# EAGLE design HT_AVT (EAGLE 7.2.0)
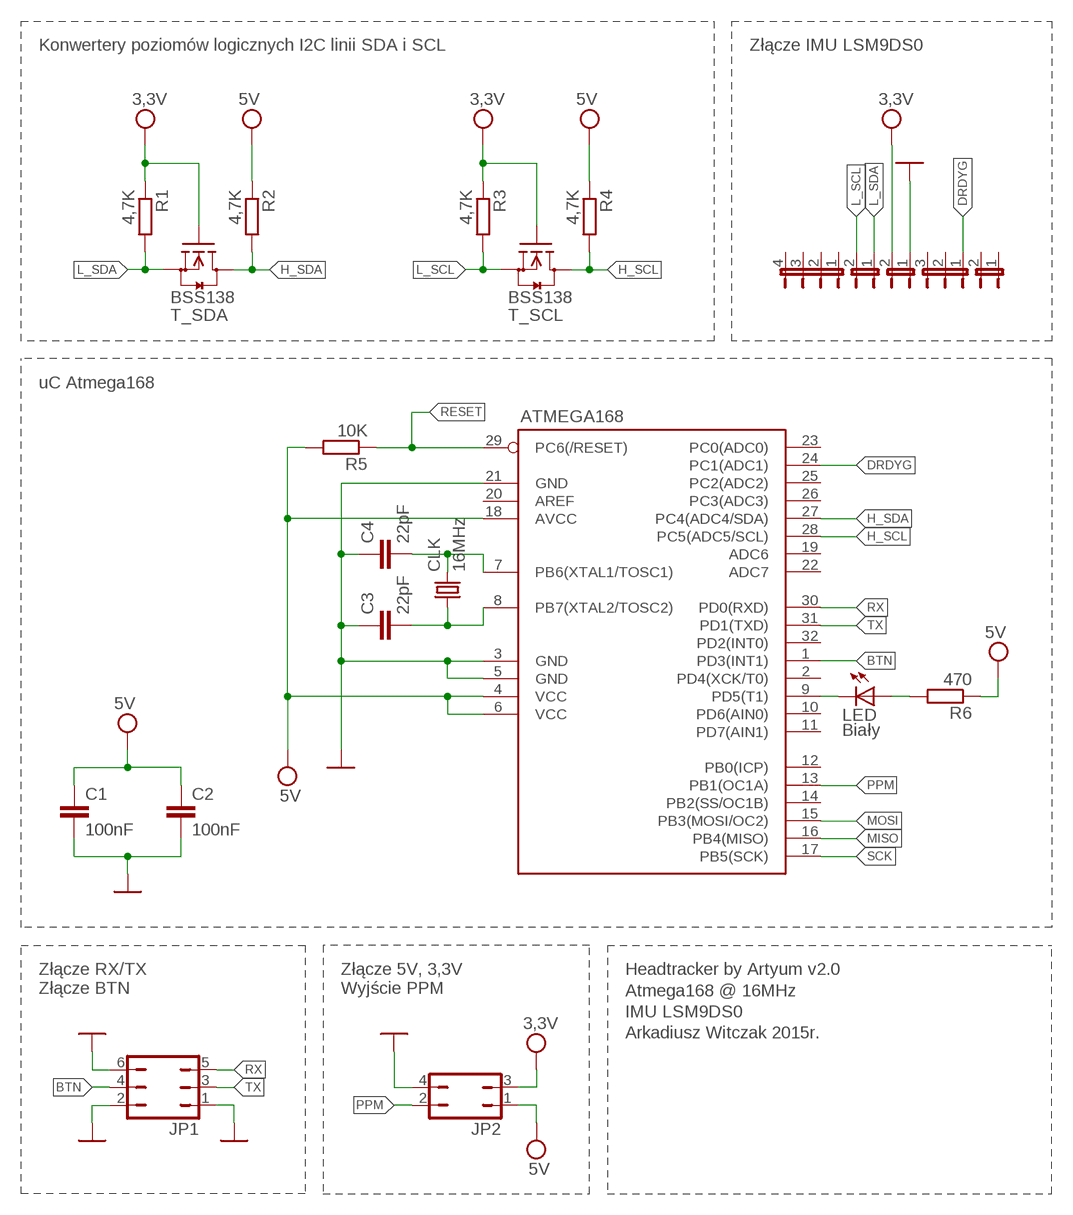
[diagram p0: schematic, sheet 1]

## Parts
ATMEGA168  MEGA8-AI  [TQFP32-08]
C1  100nF  C-EUC0805  [C0805]
C2  100nF  C-EUC0805  [C0805]
C3  22pF  C-EUC0805  [C0805]
C4  22pF  C-EUC0805  [C0805]
CLK  16MHz  CRYSTALHC49U-V  [HC49U-V]
J1  JP1E  [JP1]
J2  JP1E  [JP1]
J3  JP1E  [JP1]
J4  JP2E  [JP2]
J5  JP4E  [JP4]
JP1  JP3Q  [JP3Q]
JP2  JP2Q  [JP2Q]
LED  Biały  LEDCHIPLED_0805  [CHIPLED_0805]
R1  4,7K  R-EU_R0805  [R0805]
R2  4,7K  R-EU_R0805  [R0805]
R3  4,7K  R-EU_R0805  [R0805]
R4  4,7K  R-EU_R0805  [R0805]
R5  10K  R-EU_R0805  [R0805]
R6  470  R-EU_R0805  [R0805]
T_SCL  BSS138  [SOT23]
T_SDA  BSS138  [SOT23]

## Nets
BTN: ATMEGA168.1(PD3(INT1)) JP1.4
DRDYG: ATMEGA168.24(PC1(ADC1)) J4.1
GND: ATMEGA168.3(GND) ATMEGA168.5(GND) ATMEGA168.21(GND) C1.2 C2.2 C3.1 C4.1 J3.1 JP1.1 JP1.2 JP1.6 JP2.4
H_SCL: ATMEGA168.28(PC5(ADC5/SCL)) R4.2 T_SCL.3(D)
H_SDA: ATMEGA168.27(PC4(ADC4/SDA)) R2.2 T_SDA.3(D)
HV: ATMEGA168.4(VCC) ATMEGA168.6(VCC) ATMEGA168.18(AVCC) C1.1 C2.1 JP2.1 R2.1 R4.1 R5.2 R6.1 ; supply symbol labelled 5V
L_SCL: J2.2 R3.2 T_SCL.2(S)
L_SDA: J2.1 R1.2 T_SDA.2(S)
LV: J3.2 JP2.3 R1.1 R3.1 T_SCL.1(G) T_SDA.1(G) ; supply symbol labelled 3,3V
MISO: ATMEGA168.16(PB4(MISO))
MOSI: ATMEGA168.15(PB3(MOSI/OC2))
N$3: ATMEGA168.8(PB7(XTAL2/TOSC2)) C3.2 CLK.1
N$4: ATMEGA168.9(PD5(T1)) LED.C
N$5: ATMEGA168.7(PB6(XTAL1/TOSC1)) C4.2 CLK.2
N$8: LED.A R6.2
PPM: ATMEGA168.13(PB1(OC1A)) JP2.2
RESET: ATMEGA168.29(PC6(/RESET)) R5.1
RX: ATMEGA168.30(PD0(RXD)) JP1.5
SCK: ATMEGA168.17(PB5(SCK))
TX: ATMEGA168.31(PD1(TXD)) JP1.3
Unconnected: ATMEGA168.2(PD4(XCK/T0)) ATMEGA168.10(PD6(AIN0)) ATMEGA168.11(PD7(AIN1)) ATMEGA168.12(PB0(ICP)) ATMEGA168.14(PB2(SS/OC1B)) ATMEGA168.19(ADC6) ATMEGA168.20(AREF) ATMEGA168.22(ADC7) ATMEGA168.23(PC0(ADC0)) ATMEGA168.25(PC2(ADC2)) ATMEGA168.26(PC3(ADC3)) ATMEGA168.32(PD2(INT0)) J1.1 J1.2 J4.2 J4.3 J5.1 J5.2 J5.3 J5.4

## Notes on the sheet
- Konwertery poziomów logicznych I2C linii SDA i SCL | Złącze IMU LSM9DS0
- uC Atmega168
- Złącze RX/TX
  Złącze BTN
- Złącze 5V, 3,3V
  Wyjście PPM
- Headtracker by Artyum v2.0 
  Atmega168 @ 16MHz
  IMU LSM9DS0
  Arkadiusz Witczak 2015r.

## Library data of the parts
ATMEGA168 = atmel:MEGA8: MICROCONTROLLER 8 Kbytes FLASH, 1 kbytes SRAM, 512 bytes EEPROM, USART, 6-channel 10 bit ADC, 2-channel 8 bit ADC Pin compatible with Atmega48, ATMega88, ATMega168 Source: avr.lbr; MPN: ATMEGA8-16AU; OC_FARNELL: 9171371; OC_NEWARK: 73M8863
C1-C4 = rcl:C-EU: CAPACITOR, European symbol
CLK = crystal:CRYSTAL: CRYSTAL; OC_FARNELL: 1666969; OC_NEWARK: unknown
J1-J3 = jumper:JP1E: JUMPER
J4 = jumper:JP2E: JUMPER
J5 = jumper:JP4E: JUMPER
JP1 = jumper:JP3Q: JUMPER
JP2 = jumper:JP2Q: JUMPER
LED = led:LED: LED
R1-R6 = rcl:R-EU_: RESISTOR, European symbol
T_SCL T_SDA = m-pad-2.1:BSS138: Fairchild Semiconductors BSS138 N-Channel Logic Level Enhancement Mode Field Effect Transistor General Description: These N-Channel enhancement mode field effect transistors are produced using Fairchild's proprietary, high cell density, DMOS technology. These products have been designed to minimize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

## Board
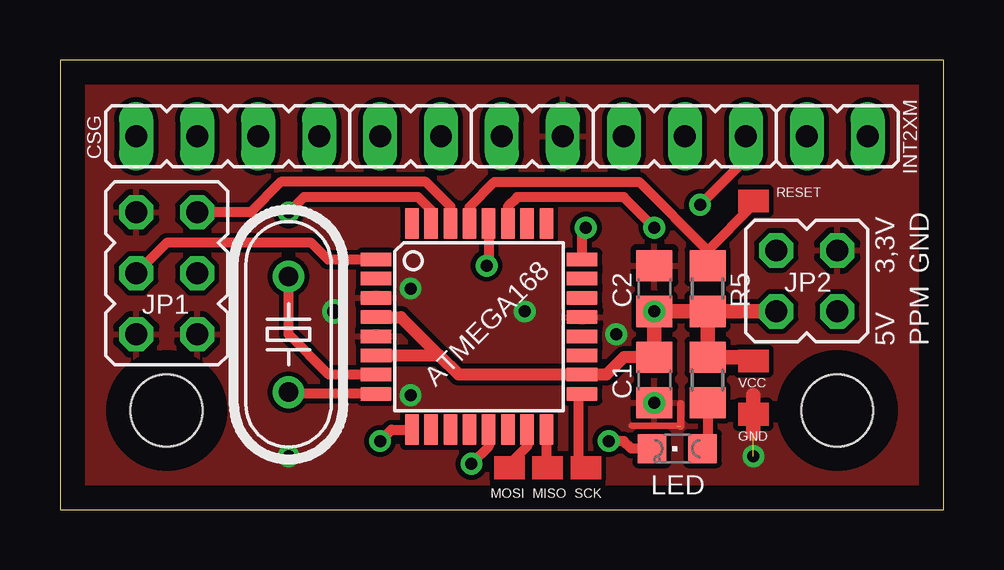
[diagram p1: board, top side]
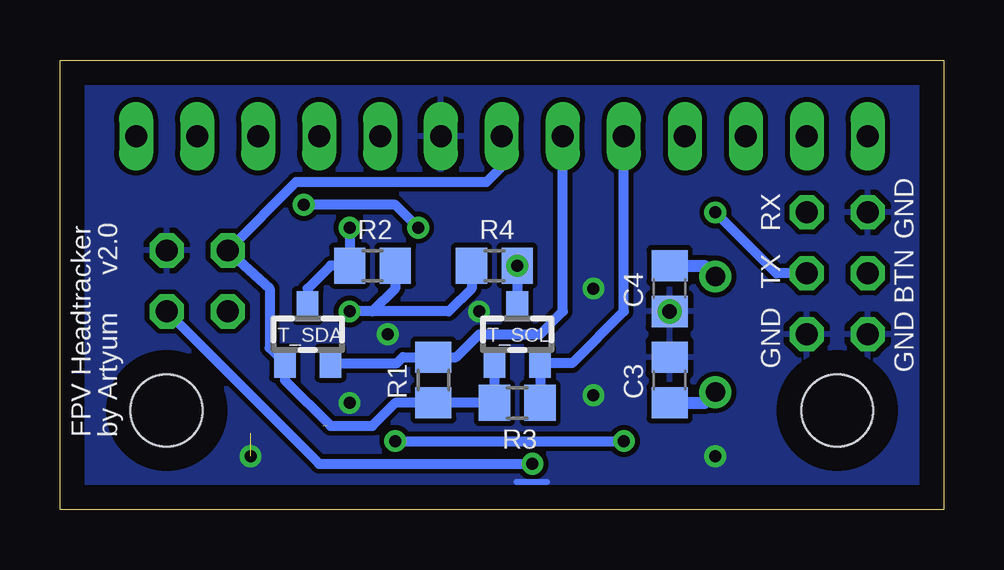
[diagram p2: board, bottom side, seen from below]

Size 36.83 x 18.73 mm. Coordinates in mm from the lower left corner, seen from the top.
Outline: 0,0 36.83,0 36.83,18.73 0,18.73 0,0
Copper layers (1*16): Top 0.035mm / dielectric 1.5mm / Bottom 0.035mm
Design rules "default": minimum track width 10mil, minimum drill 24mil, track to track 8mil, track to pad 8mil, pad to pad 8mil, via to via 8mil, smd to smd 8mil, copper to edge 40mil, drill to drill 8mil, minimum pad ring 10mil, minimum via ring 8mil, stop-mask expansion 4mil, vias tented up to drill 0mil, thermal gap 10mil
Holes 3 mm at 32.38,4.13 4.45,4.13

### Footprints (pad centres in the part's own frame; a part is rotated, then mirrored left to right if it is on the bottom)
TQFP32-08 = smd 1.27 x 0.559: 1 -4.293,2.8; 2 -4.293,2; 3 -4.293,1.2; 4 -4.293,0.4; 5 -4.293,-0.4; 6 -4.293,-1.2; 7 -4.293,-2; 8 -4.293,-2.8; 17 4.293,-2.8; 18 4.293,-2; 19 4.293,-1.2; 20 4.293,-0.4; 21 4.293,0.4; 22 4.293,1.2; 23 4.293,2; 24 4.293,2.8 | smd 0.559 x 1.27: 9 -2.8,-4.293; 10 -2,-4.293; 11 -1.2,-4.293; 12 -0.4,-4.293; 13 0.4,-4.293; 14 1.2,-4.293; 15 2,-4.293; 16 2.8,-4.293; 25 2.8,4.293; 26 2,4.293; 27 1.2,4.293; 28 0.4,4.293; 29 -0.4,4.293; 30 -1.2,4.293; 31 -2,4.293; 32 -2.8,4.293
C0805 = smd 1.3 x 1.5: 1 -0.95,0; 2 0.95,0
HC49U-V = drill 0.813: 1 -2.413,0; 2 2.413,0
JP1 = drill 0.914 long: 1 0,-1.27; 2 0,1.27
JP2 = drill 0.914 long: 1 -2.54,0; 2 0,0; 3 2.54,0
JP4 = drill 0.914 long: 1 -3.81,0; 2 -1.27,0; 3 1.27,0; 4 3.81,0
JP3Q = drill 0.914 octagon: 1 -2.54,-1.27; 2 -2.54,1.27; 3 0,-1.27; 4 0,1.27; 5 2.54,-1.27; 6 2.54,1.27
JP2Q = drill 0.914 octagon: 1 -1.27,-1.27; 2 1.27,-1.27; 3 -1.27,1.27; 4 1.27,1.27
CHIPLED_0805 = smd 1.2 x 1.2: A 0,-1.05; C 0,1.05
R0805 = smd 1.3 x 1.5: 1 -0.95,0; 2 0.95,0
SOT23 = smd 0.9 x 1.2: 1 -0.95,-1.2; 2 0.95,-1.2; 3 0,1.2

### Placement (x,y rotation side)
ATMEGA168  17.46,7.62 0 top
C1  24.77,5.4 270 top
C2  24.77,9.21 90 top
C3  11.43,5.4 270 bottom
C4  11.43,9.21 90 bottom
CLK  9.52,7.3 90 top
J1  32.38,15.56 270 top
J2  14.6,15.56 90 top
J3  19.69,15.56 90 top
J4  26.03,15.56 180 top
J5  6.98,15.56 180 top
JP1  4.45,9.84 90 top
JP2  31.12,9.53 0 top
LED  25.72,2.54 90 top
R1  21.27,5.4 90 bottom
R2  23.81,10.16 180 bottom
R3  17.78,4.45 0 bottom
R4  18.73,10.16 0 bottom
R5  26.99,9.21 270 top
R6  26.99,5.4 270 top
T_SCL  17.78,7.3 0 bottom
T_SDA  26.51,7.3 0 bottom

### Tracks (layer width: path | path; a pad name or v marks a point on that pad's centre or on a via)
BTN
  Top 0.406: ATMEGA168.1 11.17,10.42 10.48,11.11 4.45,11.11 JP1.4
DRDYG  (via drill 0.5)
  Top 0.406: v26.67,12.7 28.57,14.61 J4.1 | ATMEGA168.24 21.76,11.6 v21.91,11.75
  Bottom 0.406: v26.67,12.7 22.86,12.7 v21.91,11.75
GND  (via drill 0.5, 0.6)  (2 unrouted)
  Top 0.279: 25.72,3.49 23.81,3.49
  Top 0.305: 25.87,4.42 25.87,3.47
  Top 0.61: 28.89,4.76 28.89,3.18
  Bottom 0.254: 16.54,1.14 17.81,1.14
  other vias: 23.18,7.3 14.6,4.76 14.6,9.21 11.43,8.25 19.37,8.25 24.77,4.45 20.95,15.56 5.71,7.3 3.18,7.3 3.18,12.38 32.38,10.79 28.89,2.22 9.52,2.22
  pour Bottom: -0.95,19.68 37.78,19.68 37.78,-0.95 -0.95,-0.95
  pour Top: -0.64,19.37 37.46,19.37 37.46,-0.64 -0.64,-0.64
H_SCL  (via drill 0.5)
  Top 0.406: ATMEGA168.28 17.86,10.24 R4.2
  Bottom 0.406: R4.2 T_SCL.3
  other vias: 17.78,10.16
H_SDA  (via drill 0.5)
  Top 0.406: v24.77,11.75 23.49,13.02 19.05,13.02 18.66,12.63 ATMEGA168.27
  Bottom 0.406: v24.77,11.75 24.77,11.43 R2.2 25.56,10.16 26.51,9.21 T_SDA.3
HV  (via drill 0.5)  (1 unrouted)
  Top 0.406: R5.2
  Top 0.508: ATMEGA168.4 14.2,8.02 15.81,6.42 | 15.81,6.42 ATMEGA168.6 | 15.81,6.42 16.6,5.62 ATMEGA168.18 22.77,5.62 23.49,6.35 C1.1
  Top 0.61: JP2.1 R5.2 R6.1 | R5.2 C2.1 | C2.1 C1.1 | R6.1 | R6.1 28.73,6.35
  Bottom 0.406: R2.1 22.86,9.21 23.81,8.25 | R4.1 19.68,9.21 20.64,8.25 23.81,8.25 | 23.81,8.25 C2.1
  other vias: 24.77,8.25
L_SCL
  Bottom 0.406: J2.2 13.34,8.25 15.49,6.1 T_SCL.2 R3.2
L_SDA
  Bottom 0.406: J2.1 15.88,8.25 16.83,7.3 19.37,7.3 20.32,6.35 R1.2 22.54,6.35 22.79,6.1 T_SDA.2
LV
  Bottom 0.406: J3.2 18.42,14.29 19.05,13.65 26.99,13.65 JP2.3 28.1,9.21 28.1,6.74 T_SDA.1 27.46,5.39 25.56,3.49 23.81,3.49 22.86,4.45 R1.1 R3.1 T_SCL.1
MISO
  Top 0.406: ATMEGA168.16 20.26,1.8
MOSI
  Top 0.406: ATMEGA168.15 19.46,2.63 18.73,1.9
N$3
  Top 0.406: ATMEGA168.8 9.59,4.82 CLK.1
  Bottom 0.508: C3.2 9.97,4.45 CLK.1
N$4  (via drill 0.5)
  Top 0.406: v13.34,2.86 13.8,3.33 ATMEGA168.9 | LED.C 23.81,2.54 23.49,2.86 v22.86,2.86
  Bottom 0.406: v22.86,2.86 v13.34,2.86
N$5
  Top 0.406: ATMEGA168.7 11.21,5.62 9.52,7.3 CLK.2
  Bottom 0.508: C4.2 9.97,10.16 CLK.2
N$8
  Top 0.406: R6.2 26.99,2.76 LED.A
PPM  (via drill 0.5)
  Top 0.406: ATMEGA168.13 17.86,2.62 v17.14,1.9
  Bottom 0.406: JP2.2 26.03,1.9 v17.14,1.9
RESET
  Top 0.406: ATMEGA168.29 17.06,12.62 18.1,13.65 24.13,13.65 26.99,10.79 | R5.1 26.99,10.79 | 26.99,10.79 28.89,12.7
RX
  Top 0.406: ATMEGA168.30 16.26,12.63 15.24,13.65 9.21,13.65 7.94,12.38 JP1.5
SCK
  Top 0.406: ATMEGA168.17 21.59,4.82 21.59,1.9
TX  (via drill 0.5)
  Top 0.406: ATMEGA168.31 15.46,12.48 14.92,13.02 10.16,13.02 v9.52,12.38
  Bottom 0.406: JP1.3 6.99,9.84 v9.52,12.38
(copper drawn outside any net)
  shapes: Top area x6

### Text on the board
tNames: CSG | RESET | INT2XM | 3,3V | GND | 5V | PPM | VCC | GND | MOSI | MISO | SCK
bNames: GND | RX | TX | BTN | GND | GND | by Artyum v2.0 | FPV Headtracker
